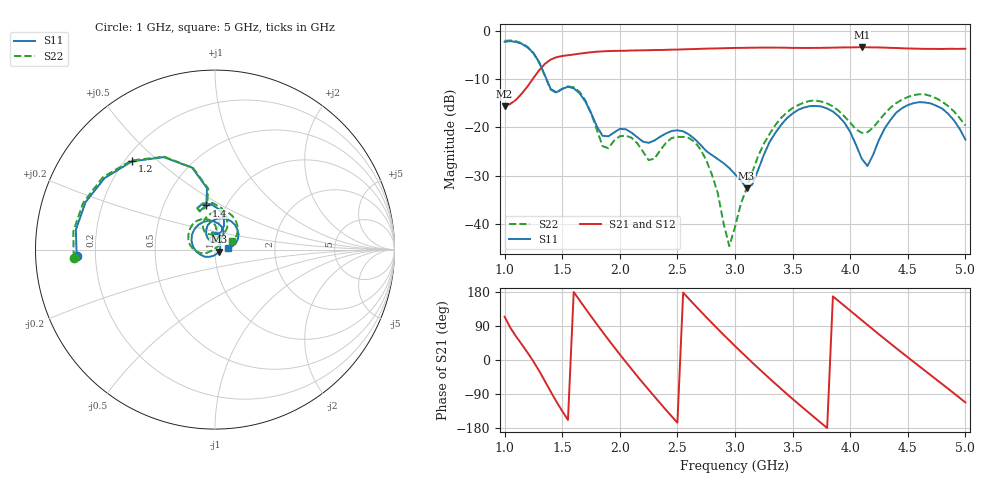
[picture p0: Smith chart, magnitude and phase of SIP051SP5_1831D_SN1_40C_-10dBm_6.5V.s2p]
# GHz  S  dB  R  50
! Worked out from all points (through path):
!   81 points, 1 GHz to 5 GHz, reference 50 ohm
!   highest |S21| = -3.38 dB at 4.1 GHz (marker M1); lowest = -15.6 dB at 1 GHz (marker M2)
!   lowest |S11| = -32.6 dB at 3.1 GHz (marker M3), VSWR 1.05, Z = 52.1 - j1.17 ohm
!   |S11| at or under -10 dB: 1.364 GHz to end of sweep
!   |S22| runs from -44.6 to -2.0 dB; largest |S21 - S12| = 0.0028
!   S11 on the Smith chart (normalised r, x): 1 GHz: 0.13, -0.02; 1.2 GHz: 0.23, +0.41; 1.4 GHz: 0.81, +0.42; 5 GHz: 1.16, +0.02
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1  -2.25 -177.3  -15.63 114.2  -15.63 114.1  -2.06 -176.7
1.2  -3.41 133.3  -11.46 19.1  -11.45 19.1  -3.34 133.2
1.3  -6.48 105.6  -8.15 -28.8  -8.14 -28.9  -6.55 105.0
1.4  -12.02 101.1  -5.94 -83.3  -5.93 -83.3  -12.16 100.4
1.55  -11.57 105.9  -5.04 -158.1  -5.04 -158.2  -11.49 105.0
1.7  -14.58 74.8  -4.57 136.5  -4.58 136.5  -14.36 69.6
1.85  -21.71 82.4  -4.24 74.3  -4.23 74.3  -23.85 73.1
2.05  -20.36 94.6  -4.12 -4.3  -4.12 -4.2  -21.71 93.4
2.2  -22.91 92.2  -4.02 -60.3  -4.03 -60.2  -24.94 84.0
2.35  -21.92 103.5  -3.96 -113.9  -3.95 -113.9  -24.76 116.4
2.6  -21.44 70.8  -3.79 161.4  -3.79 161.3  -22.19 76.8
2.8  -25.71 55.6  -3.65 97.5  -3.65 97.5  -29.76 47.1
2.95  -28.38 39.5  -3.56 51.9  -3.56 51.8  -44.56 132.2
3  -29.66 27.5  -3.53 36.9  -3.52 37.0  -40.62 -178.2
3.1  -32.56 -28.6  -3.51 7.8  -3.50 7.7  -32.64 -159.6
3.4  -19.45 -175.5  -3.48 -76.1  -3.47 -76.0  -18.02 176.7
3.7  -15.54 113.1  -3.53 -154.3  -3.53 -154.2  -14.43 122.7
3.9  -17.68 72.7  -3.45 155.4  -3.46 155.3  -16.53 92.8
4.1  -26.45 67.3  -3.38 105.1  -3.38 105.1  -21.12 97.4
4.35  -18.42 114.1  -3.52 43.2  -3.52 43.3  -15.90 114.8
4.65  -14.82 60.0  -3.73 -28.4  -3.71 -28.2  -13.15 70.9
5  -22.50 7.9  -3.70 -112.0  -3.71 -111.9  -19.59 26.4
